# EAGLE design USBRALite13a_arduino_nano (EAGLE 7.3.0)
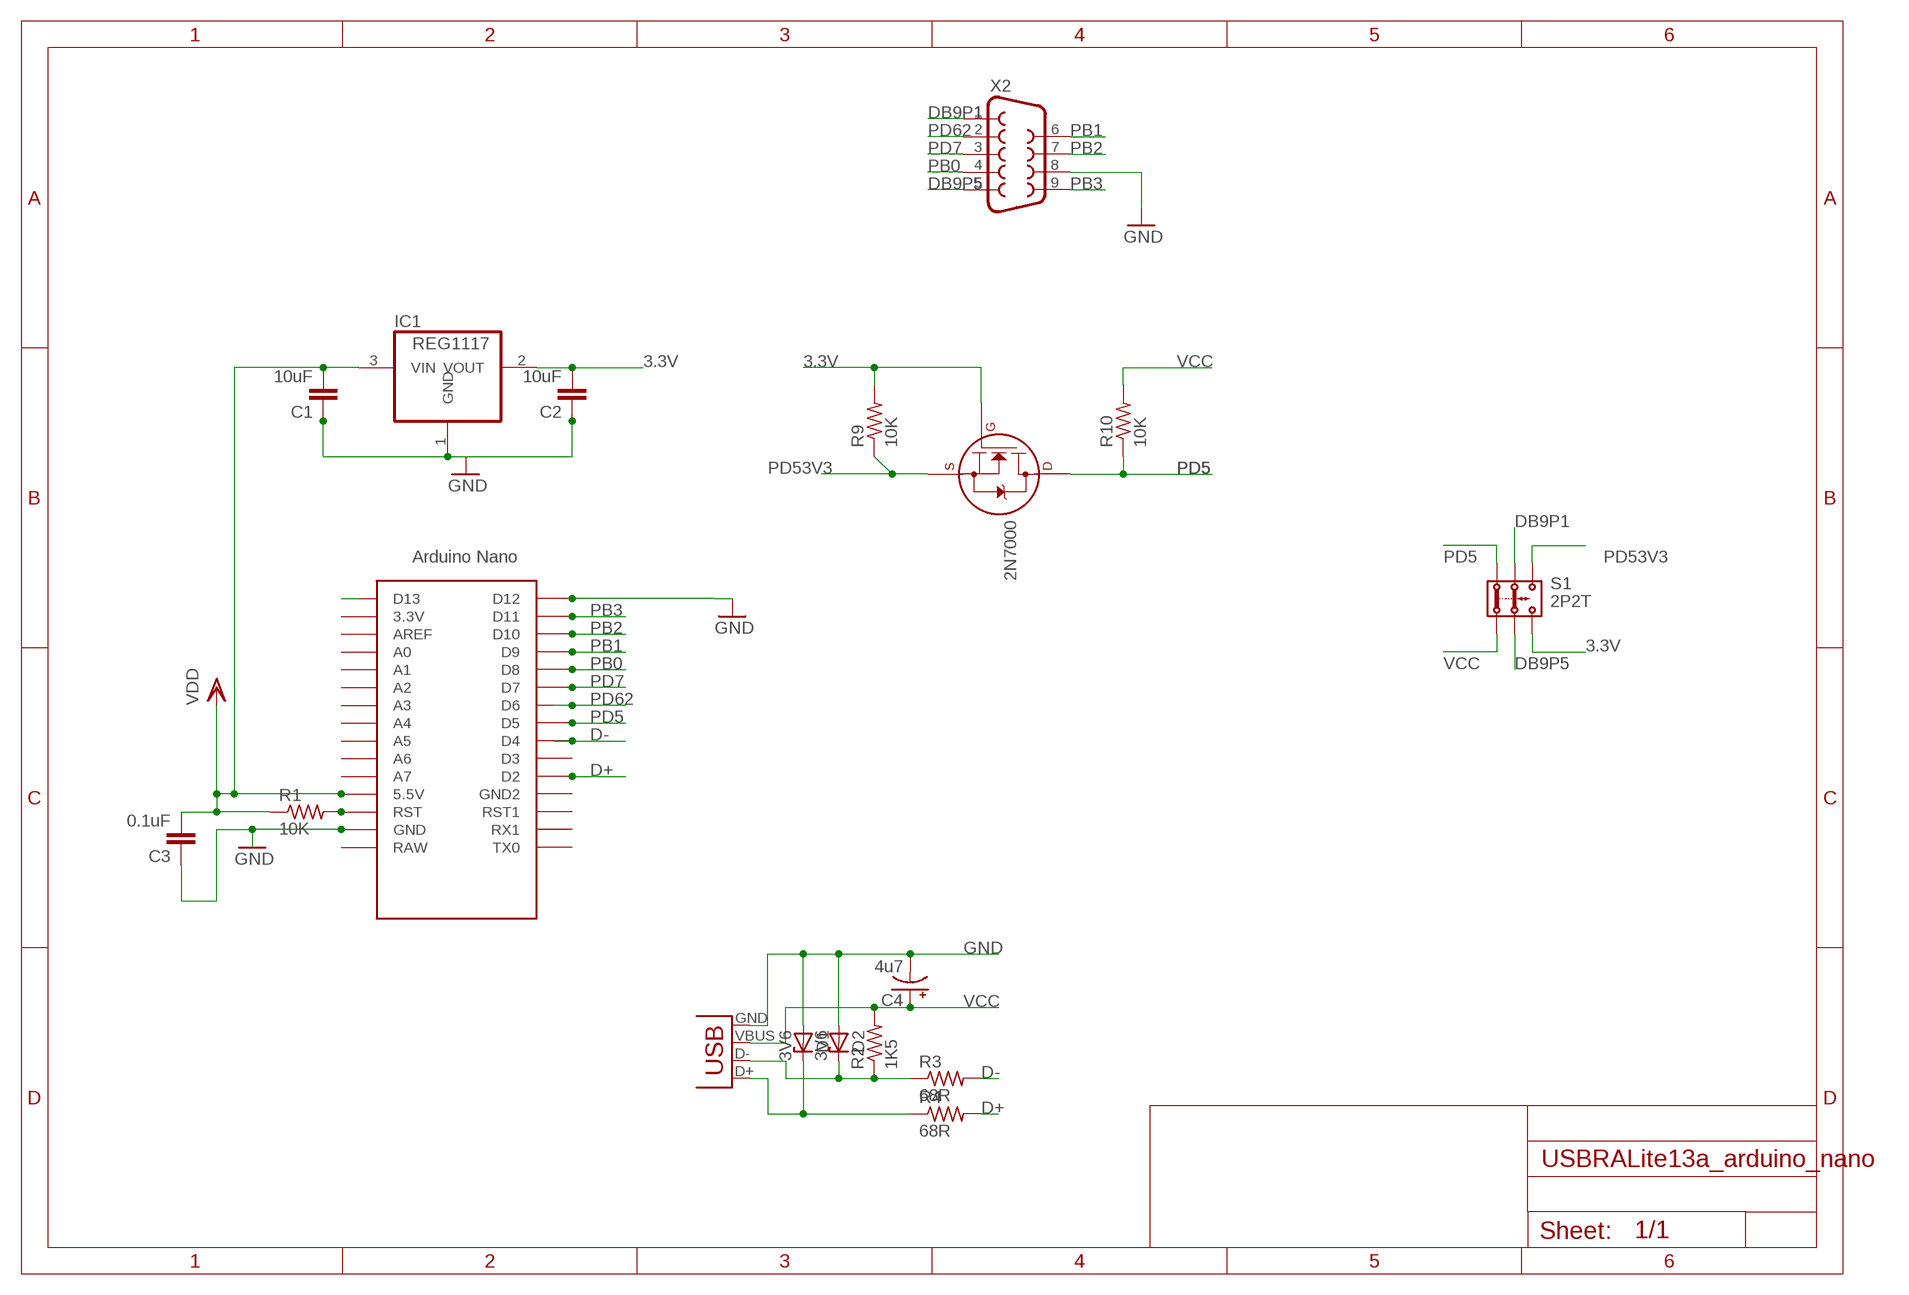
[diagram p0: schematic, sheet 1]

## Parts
2N7000  2N7000_TO92  [TO-92]
C1  10uF  C-EU050-024X044  [C050-024X044]
C2  10uF  C-EU050-024X044  [C050-024X044]
C3  0.1uF  C-EU050-024X044  [C050-024X044]
C4  4u7  CPOL-USE2.5-6  [E2,5-6]
D1  3V6  ZENER-DIODEZD-5  [ZDIO-5]
D2  3V6  ZENER-DIODEZD-5  [ZDIO-5]
IC1  REG1117  [SOT223]
R1  10K  R-US_0207/10  [0207/10]
R2  1K5  R-US_0207/10  [0207/10]
R3  68R  R-US_0207/10  [0207/10]
R4  68R  R-US_0207/10  [0207/10]
R9  10K  R-US_0207/10  [0207/10]
R10  10K  R-US_0207/10  [0207/10]
S1  2P2T  [2P2T]
U$1  NANO  [NANO]
X1  USBPTH  [USB-B-PTH]
X2  DB9MALE  [DB9_MALE]

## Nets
3.3V: 2N7000.2(G) C2.2 IC1.2(VOUT) R9.2 S1.3.2
D+: R4.2 U$1.D2
D-: R3.2 U$1.D4
DB9P1: S1.2.1 X2.1
DB9P5: S1.2.2 X2.5
GND: C1.1 C2.1 C3.1 C4.- D1.A D2.A IC1.1(GND) U$1.GND X1.GND X2.8
N$1: R1.2 U$1.RST
N$3: U$1.D12
N$4: U$1.D13
N$8: D1.C R4.1 X1.D+
N$9: D2.C R2.1 R3.1 X1.D-
PB0: U$1.D8 X2.4
PB1: U$1.D9 X2.6
PB2: U$1.D10 X2.7
PB3: U$1.D11 X2.9
PD5: 2N7000.3(D) R10.1 S1.1.1 U$1.D5
PD7: U$1.D7 X2.3
PD53V3: 2N7000.1(S) R9.1 S1.3.1
PD62: U$1.D6 X2.2
VCC: C1.2 C3.2 C4.+ IC1.3(VIN) R1.1 R2.2 R10.2 S1.1.2 U$1.5V(5.5V) X1.VBUS ; supply symbol labelled VDD
Unconnected: U$1.3.3V U$1.A0 U$1.A1 U$1.A2 U$1.A3 U$1.A4 U$1.A5 U$1.A6 U$1.A7 U$1.AREF U$1.D3 U$1.GND1(GND2) U$1.ICSP1 U$1.ICSP2 U$1.ICSP3 U$1.ICSP4 U$1.ICSP5 U$1.ICSP6 U$1.RAW U$1.RST1 U$1.RX1 U$1.TX0

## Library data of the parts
2N7000 = transistors:2N700*: 2N7000, 2N7002, NDS7002A N-channel enhancement mode MOSFET
C1-C3 = rcl:C-EU: CAPACITOR, European symbol
C4 = adafruit:CPOL-US: POLARIZED CAPACITOR, American symbol
D1 D2 = diode:ZENER-DIODE: Z-Diode
IC1 = burr-brown:REG1117: 800mA and 1A Low Dropout (LDO) Positive Regulator 1.8V, 2.5V, 2.85V, 3.3V, 5V, and Adj; MPN: REG1117; OC_FARNELL: 1097566; OC_NEWARK: 14P6981
R1-R4 R9 R10 = adafruit:R-US_: RESISTOR, American symbol
S1 = Itead_BP_110825:2P2T: BAS011
U$1 = Arduino-clone:NANO: Arduino Nano
X1 = SparkFun:USB: USB Connectors USB-B-PTH is fully proven SKU : PRT-00139 USB-miniB is fully proven SKU : PRT-00587 USB-A-PCB is untested. USB-A-H is throughly reviewed, but untested. Spark Fun Electronics SKU : PRT-00437 USB-B-SMT is throughly reviewed, but untested. Needs silkscreen touching up. USB-A-S has not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
X2 = SparkFun:DB9: DB9 Connector Standard DB9 (D-Sub 9) serial connector. Can be used for CAN bus as well as RS485 and RS232. Footprint production proven. Spark Fun Electronics SKU : PRT-00429

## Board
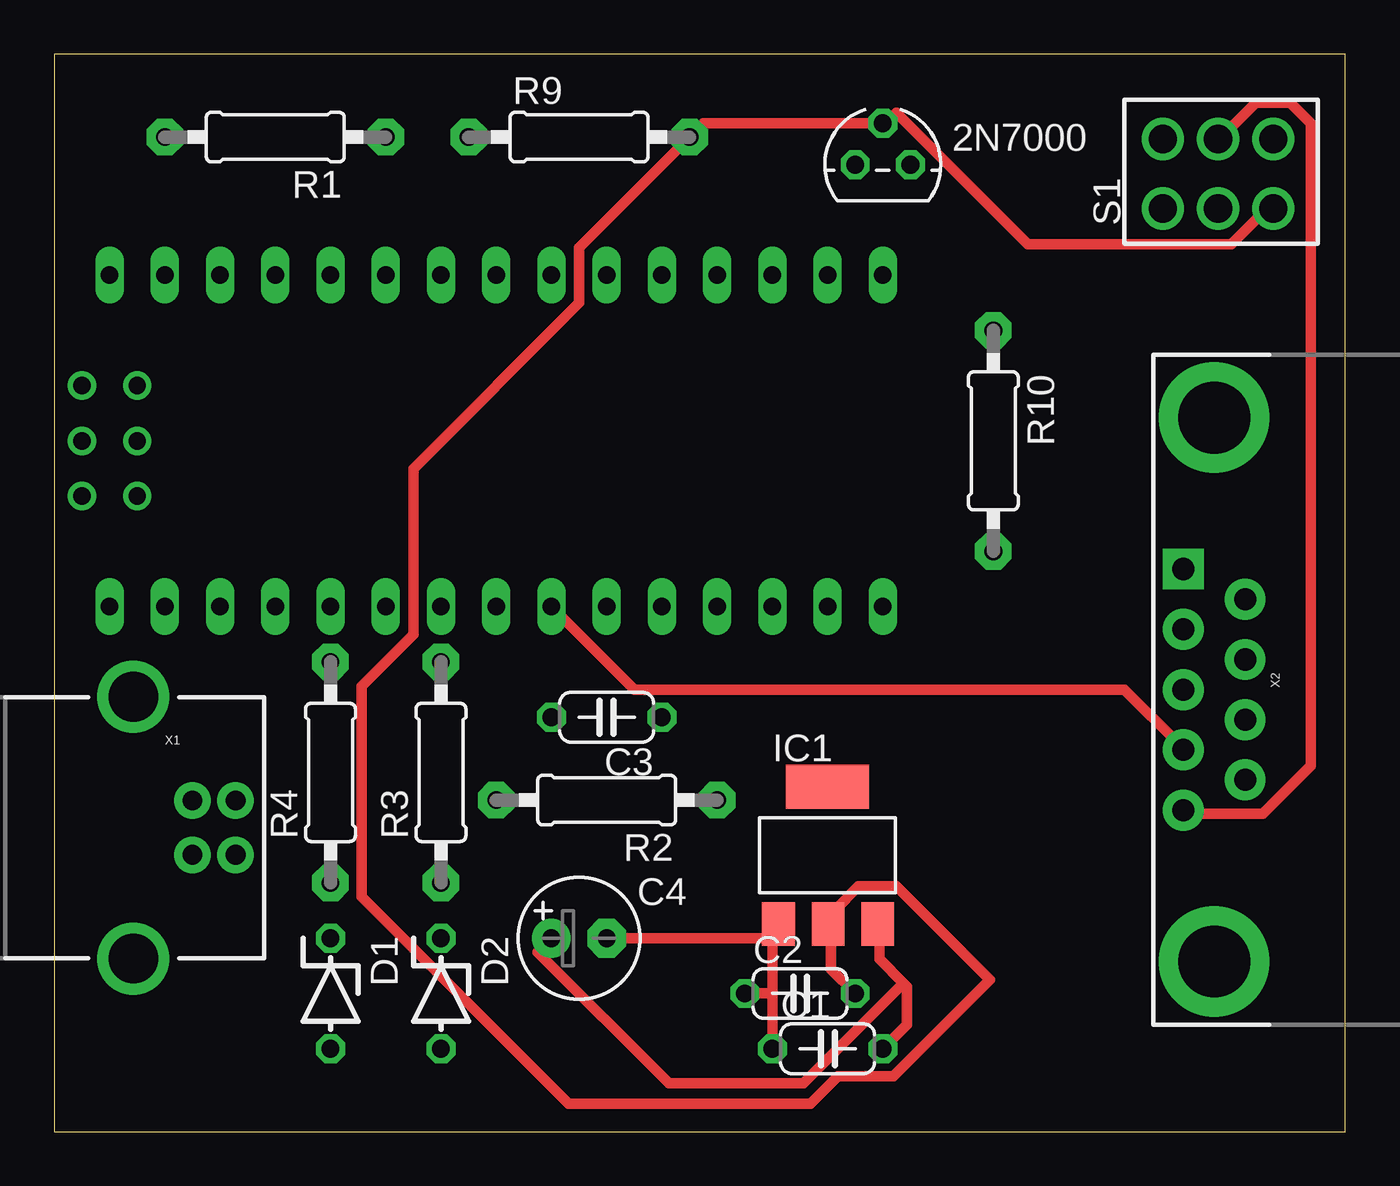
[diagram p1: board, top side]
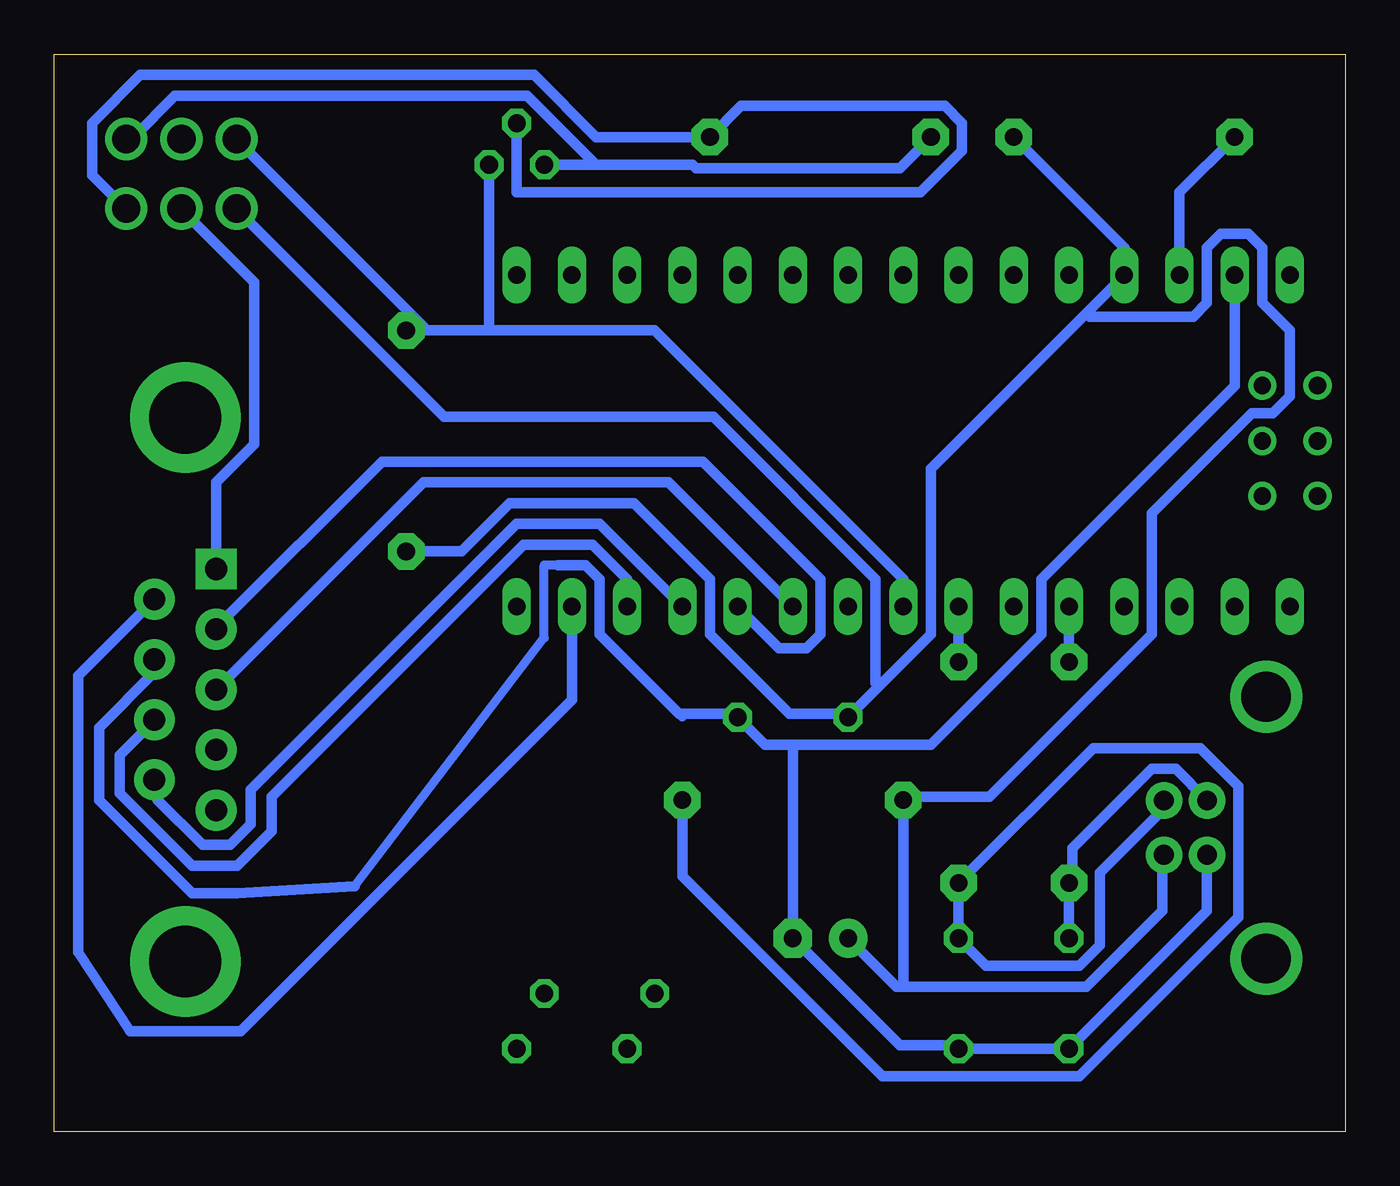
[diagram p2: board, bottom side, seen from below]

Size 59.36 x 49.52 mm. Coordinates in mm from the lower left corner, seen from the top.
Outline: 0,0 59.36,0 59.36,49.52 0,49.52 0,0
Copper layers (1*16): Top 0.035mm / dielectric 1.5mm / Bottom 0.035mm
Design rules "default *": minimum track width 19mil, minimum drill 24mil, track to track 13mil, track to pad 13mil, pad to pad 13mil, via to via 13mil, smd to smd 13mil, copper to edge 40mil, drill to drill 8mil, minimum pad ring 10mil, minimum via ring 8mil, stop-mask expansion 4mil, vias tented up to drill 0mil, thermal gap 10mil

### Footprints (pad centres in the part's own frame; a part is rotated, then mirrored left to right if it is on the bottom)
TO-92 = drill 0.813 octagon: 1 -1.27,0; 2 0,1.905; 3 1.27,0
C050-024X044 = drill 0.813 octagon: 1 -2.54,0; 2 2.54,0
E2,5-6 = drill 0.813 pad 1.778: + -1.27,0 | drill 0.813 pad 1.778 octagon: - 1.27,0
ZDIO-5 = drill 0.813 octagon: A 2.54,0; C -2.54,0
SOT223 = smd 1.499 x 2.007: 1 -2.261,-3.15; 2 0.025,-3.15; 3 2.311,-3.15 | smd 3.81 x 2.007: 4 0,3.15
0207/10 = drill 0.813 pad 1.676 octagon: 1 -5.08,0; 2 5.08,0
2P2T = drill 1.3 pad 1.93: 1.1 -3.635,-0.085; 1.2 -3.635,-3.285; 2.1 -1.095,-0.085; 2.2 -1.095,-3.285; 3.1 1.445,-0.085; 3.2 1.445,-3.285
NANO = drill 0.8 long: 3.3V -10.16,24.13; 5V -10.16,-1.27; A0 -10.16,19.05; A1 -10.16,16.51; A2 -10.16,13.97; A3 -10.16,11.43; A4 -10.16,8.89; A5 -10.16,6.35; A6 -10.16,3.81; A7 -10.16,1.27; AREF -10.16,21.59; D2 5.08,1.27; D3 5.08,3.81; D4 5.08,6.35; D5 5.08,8.89; D6 5.08,11.43; D7 5.08,13.97; D8 5.08,16.51; D9 5.08,19.05; D10 5.08,21.59; D11 5.08,24.13; D12 5.08,26.67; D13 -10.16,26.67; GND -10.16,-6.35; GND1 5.08,-1.27; RAW -10.16,-8.89; RST -10.16,-3.81; RST1 5.08,-3.81; RX1 5.08,-6.35; TX0 5.08,-8.89 | drill 0.8: ICSP1 -5.08,-10.16; ICSP2 -5.08,-7.62; ICSP3 -2.54,-10.16; ICSP4 -2.54,-7.62; ICSP5 0,-10.16; ICSP6 0,-7.62
USB-B-PTH = drill 0.914 pad 1.676: D+ 0,1.25; D- 1.981,1.25; GND 0,-1.25; VBUS 1.981,-1.25 | drill 2.286: S1 -2.718,-6.02; S2 -2.718,6.02
DB9_MALE = drill 1.016 pad 1.88: 1 5.54,-1.42; 2 2.77,-1.42; 3 0,-1.42; 4 -2.77,-1.42; 6 4.15,1.42; 7 1.38,1.42; 8 -1.38,1.42; 9 -4.15,1.42 | drill 1.016 pad 1.88 square: 5 -5.54,-1.42 | drill 3.302 pad 5.08: G1 -12.5,0; G2 12.5,0

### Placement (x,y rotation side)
2N7000  38.1,44.45 0 top
C1  35.56,3.81 0 top
C2  34.29,6.35 0 top
C3  25.4,19.05 180 top
C4  24.13,8.89 0 top
D1  12.7,6.35 270 top
D2  17.78,6.35 270 top
IC1  35.56,12.7 0 top
R1  10.16,45.72 180 top
R2  25.4,15.24 180 top
R3  17.78,16.51 90 top
R4  12.7,16.51 90 top
R9  24.13,45.72 0 top
R10  43.18,31.75 270 top
S1  54.61,45.72 0 top
U$1  11.43,29.21 270 top
X1  6.35,13.97 0 top
X2  53.34,20.32 270 top

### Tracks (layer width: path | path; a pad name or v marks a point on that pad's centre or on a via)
3.3V
  Top 0.483: C2.2 35.72,7.46 35.72,9.52 IC1.2 35.88,9.68 35.88,10.16 36.99,11.27 38.73,11.27 43.02,6.98 38.58,2.54 36.04,2.54 34.77,1.27 23.65,1.27 14.13,10.8 14.13,20.48 16.51,22.86 16.51,30.48 24.13,38.1 24.13,40.64 R9.2 29.84,46.36 2N7000.2 38.26,46.36 38.73,46.83 44.77,40.8 54.13,40.8 55.72,42.39 56.04,42.39 S1.3.2
  Bottom 0.483: 2N7000.2 38.1,43.18 19.53,43.18 17.62,45.08 17.62,46.36 18.41,47.15 27.78,47.15 R9.2 34.45,45.72 37.31,48.58 55.4,48.58 57.63,46.36 57.63,43.97 56.2,42.55 S1.3.2
D+
  Bottom 0.483: R4.2 U$1.D2
D-
  Bottom 0.483: R3.2 U$1.D4
DB9P1
  Top 0.483: X2.1 52.07,14.6 55.56,14.6 57.78,16.83 57.78,46.36 56.83,47.31 55.24,47.31 53.66,45.72 S1.2.1
DB9P5
  Bottom 0.483: X2.5 51.91,25.88 51.91,29.84 50.16,31.59 50.16,39.05 53.5,42.39 S1.2.2
GND
  Top 0.483: 33.02,6.35 C1.1 | C2.1 33.02,6.35 | 33.02,8.89 33.02,9.52 IC1.1 33.02,8.89 | C4.- 33.02,8.89 | 33.02,8.89 33.02,6.35
  Bottom 0.406: 30.48,19.05 30.48,19.21 | 45.56,11.27 36.83,22.7 36.83,26.03 36.2,26.03
  Bottom 0.483: X1.GND 6.35,10.16 D1.A D2.A 17.94,3.97 20.48,3.97 C4.- 25.4,17.78 | U$1.GND 5.08,34.29 13.97,25.4 13.97,22.86 19.05,17.78 25.4,17.78 | 25.4,17.78 26.67,17.78 C3.1 28.1,19.21 30.48,19.21 30.64,19.21 34.29,22.86 34.29,25.4 34.92,26.03 36.2,26.03 | 45.56,11.27 50.96,10.95 53.02,10.95 57.31,15.24 57.31,18.57 54.77,21.11 54.77,21.59 X2.8
N$1
  Bottom 0.483: U$1.RST 7.62,43.18 R1.2
N$8
  Bottom 0.483: D1.C R4.1 12.54,11.59 12.54,13.02 8.89,16.67 7.78,16.67 6.35,15.24 X1.D+
N$9
  Bottom 0.483: X1.D- 8.41,15.08 8.41,14.76 11.27,11.91 11.27,8.57 12.22,7.62 16.51,7.62 D2.C R3.1 11.59,17.62 6.67,17.62 4.92,15.88 4.92,9.84 12.22,2.54 21.27,2.54 30.48,11.75 R2.1
PB0
  Bottom 0.483: U$1.D8 26.04,22.23 24.77,22.23 24.13,22.86 24.13,25.4 29.53,30.8 44.29,30.8 51.91,23.18 X2.4
PB1
  Bottom 0.483: U$1.D9 34.29,27.94 38.1,27.94 50.32,15.72 50.32,14.13 51.28,13.18 52.55,13.18 54.61,15.24 54.61,16.03 X2.6
PB2
  Bottom 0.483: U$1.D10 33.02,25.4 34.61,26.99 37.78,26.99 49.37,15.4 49.37,13.81 50.96,12.22 53.02,12.22 56.36,15.56 56.36,17.3 54.77,18.89 X2.7
PB3
  Bottom 0.483: U$1.D11 35.56,19.84 50.8,4.6 55.88,4.6 58.26,8.26 58.26,20.95 54.77,24.45 X2.9
PD5
  Bottom 0.483: U$1.D5 20.32,25.4 31.75,36.83 39.37,36.83 | 39.37,36.83 R10.1 42.39,36.99 50.96,45.56 S1.1.1 | 39.37,36.83 2N7000.3
PD7
  Bottom 0.483: U$1.D7 31.11,29.84 42.39,29.84 X2.3
PD53V3
  Bottom 0.483: 34.61,44.45 30,44.45 29.84,44.29 20.48,44.29 R9.1 | 34.61,44.45 2N7000.1 | S1.3.1 56.04,45.72 55.72,45.72 53.82,47.62 37.62,47.62 34.61,44.61 34.61,44.45
PD62
  Top 0.483: U$1.D6 26.67,20.32 49.21,20.32 51.75,17.78 X2.2
VCC
  Top 0.483: 39.05,6.83 39.21,6.67 39.21,4.92 C1.2 | 39.05,6.83 37.94,7.94 37.94,9.52 IC1.3 | 39.05,6.83 34.45,2.22 28.26,2.22 22.23,8.26 C4.+
  Bottom 0.483: 20.32,6.67 20.64,6.67 C4.+ | 20.32,6.67 11.91,6.67 8.41,10.16 8.41,12.7 X1.VBUS | 20.32,6.67 R2.2 20.16,15.4 16.35,15.4 8.89,22.86 8.89,28.42 4.29,33.02 3.33,33.02 2.54,33.81 2.54,36.83 3.81,38.1 3.81,40.64 4.45,41.28 5.71,41.28 6.35,40.64 6.35,38.1 6.99,37.47 11.75,37.47 11.91,37.62 | R1.1 10.16,40.64 U$1.5V 11.91,37.62 | 21.43,20.48 19.05,22.86 19.05,30.48 11.91,37.62 | 21.43,20.48 C3.2 23.02,19.21 25.56,19.21 29.21,22.86 29.21,25.4 32.7,28.89 38.42,28.89 40.64,26.67 R10.2 | S1.1.2 50.96,42.39 41.43,32.86 29.05,32.86 21.59,25.4 21.59,20.64 21.43,20.48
